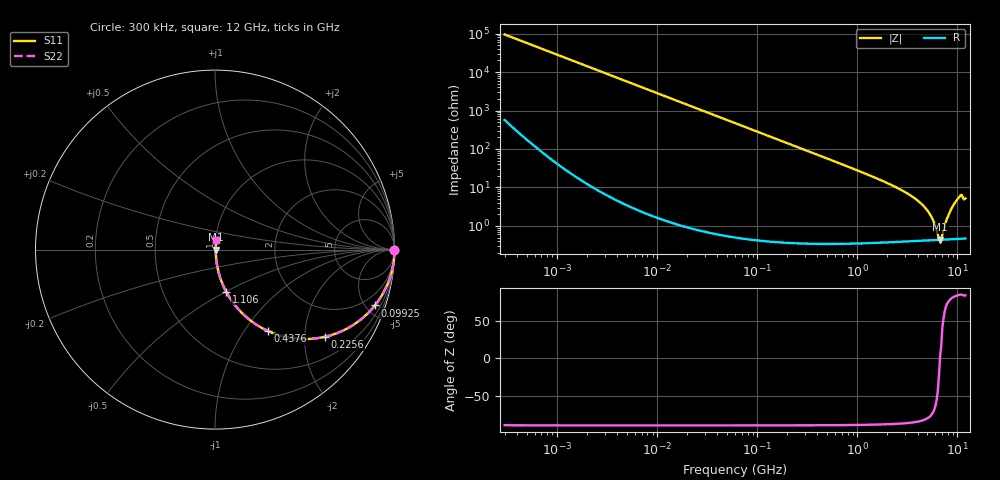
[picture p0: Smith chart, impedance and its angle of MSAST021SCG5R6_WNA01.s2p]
! MSAST021SCG5R6_WNA01  S-PARAMETER MODEL  ( General Type )
! Model Generated by TAIYO YUDEN Corporation (http://www.ty-top.com)
! Version 2.0
! TAIYO YUDEN Control No. 181101
! Copyright(c) 2015 TAIYO YUDEN CO.,LTD. All Rights Reserved.
! Product Description (link to TY-COMPAS)
! https://ds.yuden.co.jp/TYCOMPAS/or/detail?pn=MSAST021SCG5R6CWNA01&u=M
! Products Name : Multilayer Ceramic Capacitors
! Characteristics :
!  Capacitance : 5.6 pF , Rated Voltage : 25V , TCC : CG / C0G
!  Case Size : 0.25 x 0.125 / 0.0098 x 0.0049 [mm/inch] , Thickness : 0.125 / 0.0049 [mm/inch]
!  (Conditions: Temperature = 25 degC , DC Bias Current/Voltage = 0A / 0V)
! External Node Assignments :
!  1  o---| |---o  2
! GND o---------o GND
! Frequency Range : 0.3MHz  -  12000MHz  [ 401 STEP ]
# MHz S RI R 50
! Freq[MHz].  S11 Real  S11 Imag  S21 Real  S21 Imag  S12 Real  S12 Imag  S22 Real  S22 Imag
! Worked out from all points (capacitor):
!   401 points, 300 kHz to 12 GHz, reference 50 ohm
!   read as one part in series: C = 5.6 pF near 316.3 kHz
!   lowest |Z| = 438 mohm at 6.7 GHz (marker M1)
!   series resonance near 6.688 GHz, so ESL is about 100 pH
!   S11 on the Smith chart (normalised r, x): 300 kHz: open; 99.25 MHz: 1.01, -5.73; 225.6 MHz: 1.01, -2.52; 437.6 MHz: 1.01, -1.29; 1.106 GHz: 1.01, -0.50; 12 GHz: 1.01, +0.10
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0.3  1 -0.00106  7.44e-06 0.00106  7.44e-06 0.00106  1 -0.00106
1.769972  1 -0.00623  4.46e-05 0.00623  4.46e-05 0.00623  1 -0.00623
10.44266  0.9986 -0.0367  0.00137 0.0367  0.00137 0.0367  0.9986 -0.0367
60  0.9571 -0.202  0.0429 0.202  0.0429 0.202  0.9571 -0.202
99.25425  0.8909 -0.311  0.1091 0.311  0.1091 0.311  0.8909 -0.311
225.6362  0.6125 -0.4858  0.3875 0.4858  0.3875 0.4858  0.6125 -0.4858
353.9943  0.3911 -0.4858  0.6089 0.4858  0.6089 0.4858  0.3911 -0.4858
437.5599  0.2959 -0.4538  0.7041 0.4538  0.7041 0.4538  0.2959 -0.4538
686.4755  0.1458 -0.3487  0.8542 0.3487  0.8542 0.3487  0.1458 -0.3487
1105.905  0.0617 -0.2337  0.9383 0.2337  0.9383 0.2337  0.0617 -0.2337
2088.533  0.0184 -0.1201  0.9816 0.1201  0.9816 0.1201  0.0184 -0.1201
3276.641  0.00823 -0.0651  0.9918 0.0651  0.9918 0.0651  0.00823 -0.0651
4502.883  0.0053 -0.0341  0.9947 0.0341  0.9947 0.0341  0.0053 -0.0341
5420.343  0.00455 -0.0177  0.9954 0.0177  0.9954 0.0177  0.00455 -0.0177
5868.704  0.0044 -0.0109  0.9956 0.0109  0.9956 0.0109  0.0044 -0.0109
6354.153  0.00434 -0.00419  0.9957 0.00419  0.9957 0.00419  0.00434 -0.00419
6699.894  0.00435 0.000144  0.9956 -0.000144  0.9956 -0.000144  0.00435 0.000144
7064.448  0.0044 0.00385  0.9956 -0.00385  0.9956 -0.00385  0.0044 0.00385
8281.503  0.0049 0.0205  0.9951 -0.0205  0.9951 -0.0205  0.0049 0.0205
9454.42  0.00612 0.0395  0.9939 -0.0395  0.9939 -0.0395  0.00612 0.0395
10511.28  0.00781 0.0564  0.9922 -0.0564  0.9922 -0.0564  0.00781 0.0564
12000  0.0073 0.051  0.9927 -0.051  0.9927 -0.051  0.0073 0.051
